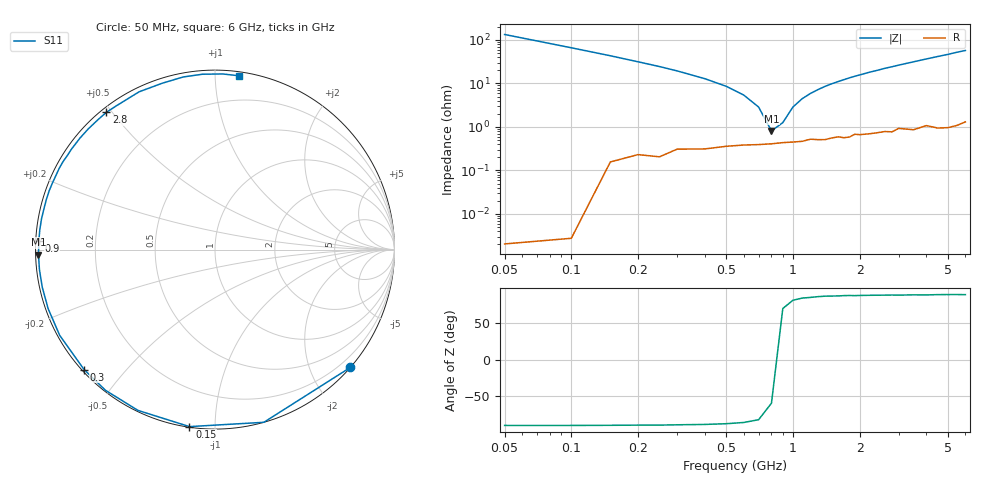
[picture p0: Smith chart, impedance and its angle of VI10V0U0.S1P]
! Infineon Technologies  Discrete & RF Semiconductors
! BB 804
! Si Tuning Diode in SOT23
! VR = 10 V
! S-Parameters:  July  1999
# GHz  S  MA  R  50
!  f  S11
! GHz  MAG  ANG
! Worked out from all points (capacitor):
!   34 points, 50 MHz to 6 GHz, reference 50 ohm
!   read as one part to ground: C = 23.7 pF near 50 MHz
!   lowest |Z| = 809 mohm at 800 MHz (marker M1)
!   series resonance near 837.2 MHz, so ESL is about 1.5 nH
!   S11 on the Smith chart (normalised r, x): 50 MHz: 0.00, -2.67; 150 MHz: 0.00, -0.87; 300 MHz: 0.01, -0.39; 900 MHz: 0.01, +0.02; 2.8 GHz: 0.02, +0.48; 6 GHz: 0.03, +1.15
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0.05  1 -41.0
0.1  1 -74.2
0.15  0.9964 -98.2
0.2  0.9934 -115.6
0.25  0.9934 -127.9
0.3  0.9893 -137.5
0.4  0.9884 -151.1
0.5  0.9862 -160.5
0.6  0.9849 -167.7
0.7  0.9845 -173.5
0.8  0.9838 -178.4
0.9  0.9827 177.3
1.1  0.9817 169.9
1.2  0.9796 166.6
1.4  0.9803 160.5
1.6  0.9777 155.1
1.9  0.9753 147.4
2.2  0.9757 140.5
2.4  0.975 136.4
2.6  0.9741 132.0
2.8  0.9754 128.3
3  0.9714 124.4
3.5  0.9756 115.7
4  0.9724 107.6
4.5  0.978 100.4
5  0.9796 94.1
5.5  0.9795 87.5
6  0.9777 82.2
